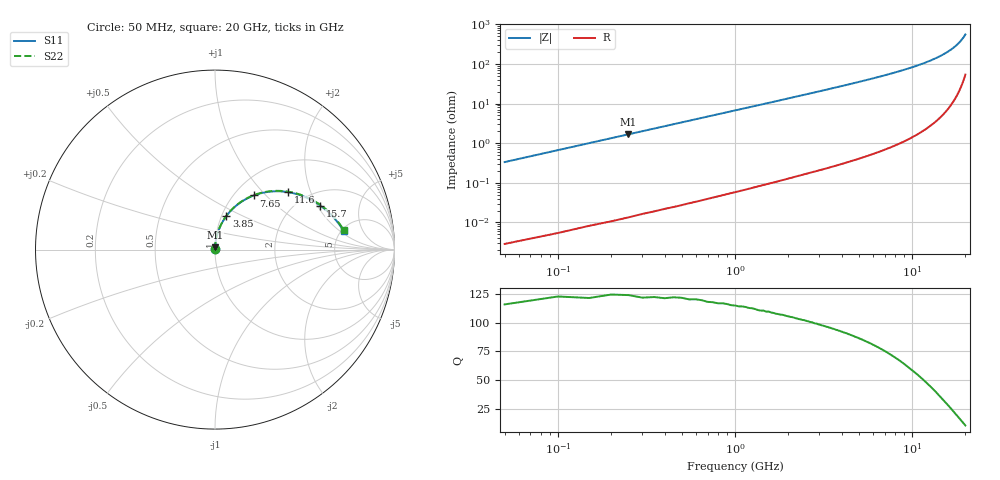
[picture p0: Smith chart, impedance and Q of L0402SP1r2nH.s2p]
!	AVX Thin Film Operation
!	Date:		5 January 2004
!	Description: 	Accu-L®  L0402 Series Thin Film RF Inductors
!	Part Number:	L04021R2AHLTR
!	50 MHz-20GHz Serial Measurements
#	mhz	S	db	R	50
!	S11	S11	S21	S21	S12	S12	S22	S22
!	dB	Phase	dB	Phase	dB	Phase	dB	Phase
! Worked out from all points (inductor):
!   400 points, 50 MHz to 20 GHz, reference 50 ohm
!   read as 1/Y11, port 2 shorted: L = 1.06 nH near 150 MHz
!   highest Q = 122 at 250 MHz (marker M1), where L = 1.06 nH
!   S11 on the Smith chart (normalised r, x): 50 MHz: 1.00, +0.01; 3.85 GHz: 1.05, +0.41; 7.65 GHz: 1.22, +0.86; 11.6 GHz: 1.62, +1.42; 15.7 GHz: 2.58, +2.13; 20 GHz: 5.27, +2.27
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50  -51.69 89.2  -0.00 -0.2  -0.00 -0.2  -51.69 89.2
100  -45.66 89.0  -0.00 -0.5  -0.00 -0.5  -45.66 89.0
150  -42.14 88.7  -0.00 -0.7  -0.00 -0.7  -42.14 88.7
200  -39.64 88.5  -0.00 -0.9  -0.00 -0.9  -39.64 88.5
250  -37.70 88.2  -0.00 -1.2  -0.00 -1.2  -37.70 88.3
400  -33.62 87.5  -0.00 -1.9  -0.00 -1.9  -33.62 87.5
600  -30.10 86.6  -0.01 -2.8  -0.01 -2.8  -30.10 86.6
850  -27.08 85.4  -0.01 -4.0  -0.01 -4.0  -27.08 85.4
1200  -24.09 83.7  -0.02 -5.6  -0.02 -5.6  -24.09 83.8
1600  -21.60 81.9  -0.04 -7.4  -0.04 -7.4  -21.60 81.9
2100  -19.26 79.5  -0.06 -9.8  -0.06 -9.8  -19.26 79.6
3400  -15.15 73.4  -0.15 -15.8  -0.15 -15.8  -15.15 73.6
3850  -14.11 71.4  -0.20 -17.8  -0.20 -17.8  -14.11 71.5
5150  -11.71 65.4  -0.34 -23.7  -0.34 -23.7  -11.71 65.6
6700  -9.62 58.5  -0.55 -30.5  -0.55 -30.5  -9.62 58.8
7650  -8.60 54.3  -0.70 -34.6  -0.70 -34.6  -8.60 54.7
10050  -6.64 44.2  -1.14 -44.6  -1.14 -44.6  -6.64 44.6
11600  -5.69 38.0  -1.46 -50.7  -1.46 -50.7  -5.69 38.5
13350  -4.83 31.3  -1.86 -57.3  -1.86 -57.3  -4.83 31.8
15700  -3.93 22.6  -2.42 -65.8  -2.42 -65.8  -3.93 23.2
16700  -3.61 19.1  -2.66 -69.2  -2.66 -69.2  -3.61 19.7
20000  -2.79 8.1  -3.50 -79.9  -3.50 -79.9  -2.79 8.8
